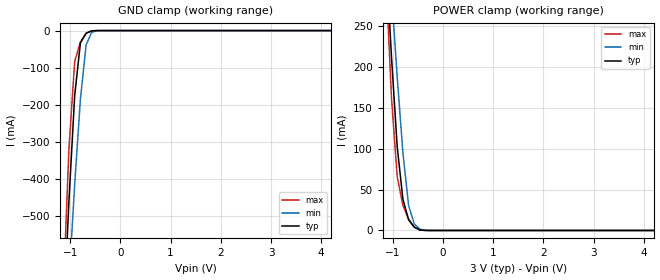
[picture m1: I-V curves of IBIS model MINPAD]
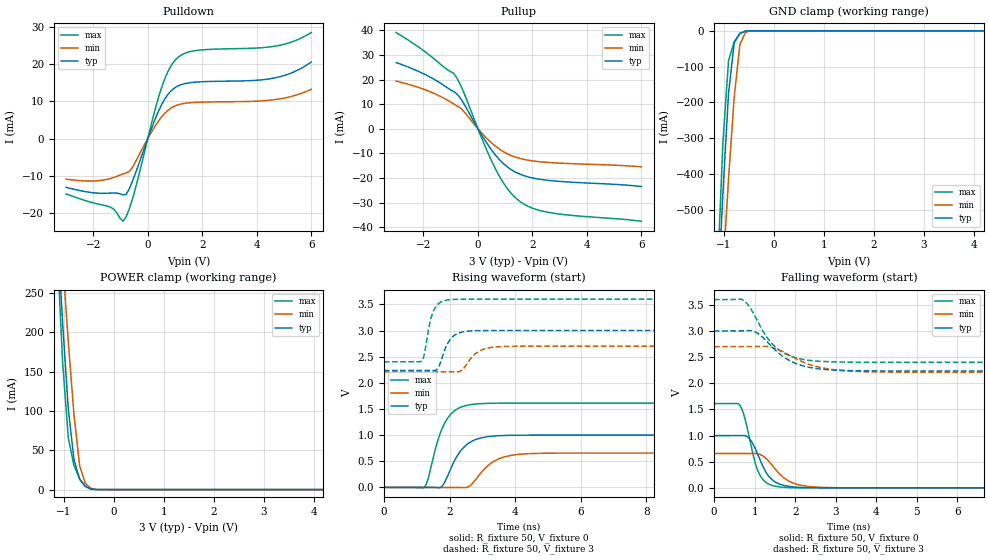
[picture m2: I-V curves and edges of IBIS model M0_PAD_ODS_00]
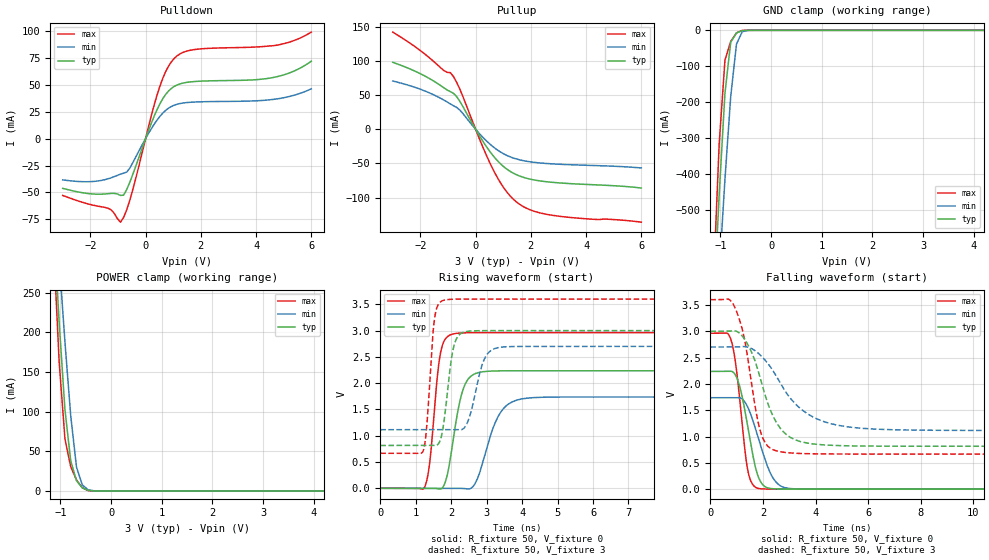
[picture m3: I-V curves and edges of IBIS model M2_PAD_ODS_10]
| Created by SiliconSmart  O-2018.09-SP2-3
[IBIS Ver]   4.0
[File Name]   as34b32bc_3p0_rev1p4.ibs
[File Rev]   1.4
[Date]   Thursday Mar 21 2024
|[Source]   Avalanche Team
|[Notes]   Generated IBIS models from Silicon Smart
|[Rev 1.0]  Initial Release based on extracted netlist
|   Characterization
|[Rev 1.1]  Recharacterization with Hspice, run in high accuracy mode
|[Rev 1.2]  Recharacterization with Hspice, parameters aligned with
|   datasheet
|[Rev 1.3]  Recharacterization with Hspice, run with updated VIH/VIL
|   in parallel with datasheet rev X.7
|[Rev 1.4]  Update the pin to the package pinout assignment
|[Disclaimer]   THE MODEL LIBRARIES ARE PROVIDED AS IS.
|[Copyright]   Copyright 2019, Avalanche Technology., All Rights Reserved
[Component]   AS304GB32_BGA
[Manufacturer] Avalanche Technology
| CONTENT :
| This file contains IBIS MODEL for PSRAM device
| AS304GB32
| USAGE :
| The models are derived for the 2.7V to 3.6V I/O Operation.
| Temperatures for model generation: typ: 25, max: -40, min: 125
| Voltages : typ: 3.0V, min: 2.7V, max: 3.6V
| PACKAGES SUPPORTED :
| 142-ball FBGA (15mm x 17mm)
| VERIFICATION
| Errors  : 0
| Warnings: 16
| All warnings due to non-monotonic data:
[Package]
R_pkg 0   0   0
L_pkg 0   0   0
C_pkg 0   0   0
[Pin]   signal_name   model_name   R_pin   L_pin   C_pin
P8   E#   MINPAD   0.254	7.307E-9	1.178E-12
P7   G#   MINPAD   0.243	7.052E-9	1.094E-12
J2   CR#   MINPAD   0.547	10.386E-9	1.789E-12
K3   PG#   MINPAD   0.451	10.329E-9	1.676E-12
M8   W#   MINPAD   0.377	9.020E-9	1.417E-12
M2   ADDR_26   MINPAD   0.425	9.037E-9	1.604E-12
L4   ADDR_25   MINPAD   0.419	9.644E-9	1.527E-12
K13   ADDR_24   MINPAD   0.495	9.978E-9	1.745E-12
M3   ADDR_23   MINPAD   0.371	9.313E-9	1.466E-12
L3   ADDR_22   MINPAD   0.412	9.753E-9	1.540E-12
M7   ADDR_21   MINPAD   0.368	8.765E-9	1.384E-12
P12   ADDR_20   MINPAD   0.287	8.287E-9	1.639E-12
L12   ADDR_19   MINPAD   0.424	10.320E-9	1.620E-12
N11   ADDR_18   MINPAD   0.338	8.691E-9	1.470E-12
N6   ADDR_17   MINPAD   0.309	8.196E-9	1.279E-12
P6   ADDR_16   MINPAD   0.256	7.462E-9	1.204E-12
L13   ADDR_15   MINPAD   0.463	10.719E-9	1.740E-12
M13   ADDR_14   MINPAD   0.421	10.290E-9	1.689E-12
P10   ADDR_13   MINPAD   0.262	7.671E-9	1.349E-12
N10   ADDR_12   MINPAD   0.340	8.540E-9	1.360E-12
M12   ADDR_11   MINPAD   0.402	9.876E-9	1.604E-12
N13   ADDR_10   MINPAD   0.399	9.819E-9	1.696E-12
L11   ADDR_9   MINPAD   0.443	9.732E-9	1.569E-12
M11   ADDR_8   MINPAD   0.436	9.682E-9	1.671E-12
P5   ADDR_7   MINPAD   0.253	7.464E-9	1.277E-12
P3   ADDR_6   MINPAD   0.279	8.031E-9	1.557E-12
N5   ADDR_5   MINPAD   0.313	8.320E-9	1.359E-12
N4   ADDR_4   MINPAD   0.329	8.138E-9	1.428E-12
M4   ADDR_3   MINPAD   0.379	8.543E-9	1.406E-12
N2   ADDR_2   MINPAD   0.378	9.572E-9	1.637E-12
N9   ADDR_1   MINPAD   0.315	8.416E-9	1.305E-12
M9   ADDR_0   MINPAD   0.403	9.225E-9	1.473E-12
E2   DQ_31   MIOPAD   0.365	8.798E-9	1.454E-12
F2   DQ_30   MIOPAD   0.418	9.057E-9	1.576E-12
D2   DQ_29   MIOPAD   0.358	8.697E-9	1.520E-12
E3   DQ_28   MIOPAD   0.348	8.812E-9	1.441E-12
E12   DQ_27   MIOPAD   0.327	8.506E-9	1.443E-12
D10   DQ_26   MIOPAD   0.309	7.715E-9	1.264E-12
C9   DQ_25   MIOPAD   0.279	7.395E-9	1.219E-12
C7   DQ_24   MIOPAD   0.252	6.802E-9	1.108E-12
G4   DQ_23   MIOPAD   0.455	10.071E-9	1.775E-12
G3   DQ_22   MIOPAD   0.457	10.100E-9	1.750E-12
F13   DQ_21   MIOPAD   0.377	9.387E-9	1.566E-12
D13   DQ_20   MIOPAD   0.295	8.231E-9	1.460E-12
C10   DQ_19   MIOPAD   0.293	7.553E-9	1.298E-12
E8   DQ_18   MIOPAD   0.393	8.323E-9	1.436E-12
F6   DQ_17   MIOPAD   0.425	8.913E-9	1.517E-12
E5   DQ_16   MIOPAD   0.379	8.982E-9	1.460E-12
E13   DQ_15   MIOPAD   0.363	8.555E-9	1.474E-12
G11   DQ_14   MIOPAD   0.475	9.536E-9	1.630E-12
E10   DQ_13   MIOPAD   0.404	8.563E-9	1.453E-12
F9   DQ_12   MIOPAD   0.409	9.347E-9	1.513E-12
C8   DQ_11   MIOPAD   0.257	6.782E-9	1.111E-12
C6   DQ_10   MIOPAD   0.238	7.000E-9	1.114E-12
D6   DQ_9   MIOPAD   0.292	7.776E-9	1.248E-12
D4   DQ_8   MIOPAD   0.305	7.782E-9	1.343E-12
G12   DQ_7   MIOPAD   0.502	10.055E-9	1.687E-12
C12   DQ_6   MIOPAD   0.275	7.857E-9	1.346E-12
D11   DQ_5   MIOPAD   0.286	7.835E-9	1.360E-12
D9   DQ_4   MIOPAD   0.306	8.035E-9	1.299E-12
E7   DQ_3   MIOPAD   0.384	8.178E-9	1.375E-12
C5   DQ_2   MIOPAD   0.231	6.786E-9	1.150E-12
D5   DQ_1   MIOPAD   0.307	7.698E-9	1.346E-12
C3   DQ_0   MIOPAD   0.267	7.420E-9	1.241E-12
G13   INT#   MIOPAD   0.480	10.704E-9	1.759E-12
F10   VSSIO   GND   NA   NA   NA
L10   VSSIO   GND   NA   NA   NA
E9   VSSIO   GND   NA   NA   NA
L9   VSSIO   GND   NA   NA   NA
F8   VSSIO   GND   NA   NA   NA
L8   VSSIO   GND   NA   NA   NA
F7   VSSIO   GND   NA   NA   NA
L7   VSSIO   GND   NA   NA   NA
E6   VSSIO   GND   NA   NA   NA
L6   VSSIO   GND   NA   NA   NA
G5   VSSIO   GND   NA   NA   NA
A14   VSS   GND   NA   NA   NA
B14   VSS   GND   NA   NA   NA
C14   VSS   GND   NA   NA   NA
H13   VSS   GND   NA   NA   NA
R14   VSS   GND   NA   NA   NA
T14   VSS   GND   NA   NA   NA
A13   VSS   GND   NA   NA   NA
T13   VSS   GND   NA   NA   NA
A12   VSS   GND   NA   NA   NA
G10   VSS   GND   NA   NA   NA
H10   VSS   GND   NA   NA   NA
J10   VSS   GND   NA   NA   NA
K10   VSS   GND   NA   NA   NA
F5   VSS   GND   NA   NA   NA
L5   VSS   GND   NA   NA   NA
A2   VSS   GND   NA   NA   NA
T2   VSS   GND   NA   NA   NA
A1   VSS   GND   NA   NA   NA
B1   VSS   GND   NA   NA   NA
R1   VSS   GND   NA   NA   NA
T1   VSS   GND   NA   NA   NA
F12   VCCIO   POWER   NA   NA   NA
J12   VCCIO   POWER   NA   NA   NA
E11   VCCIO   POWER   NA   NA   NA
M10   VCCIO   POWER   NA   NA   NA
D8   VCCIO   POWER   NA   NA   NA
N8   VCCIO   POWER   NA   NA   NA
D7   VCCIO   POWER   NA   NA   NA
N7   VCCIO   POWER   NA   NA   NA
M5   VCCIO   POWER   NA   NA   NA
E4   VCCIO   POWER   NA   NA   NA
F3   VCCIO   POWER   NA   NA   NA
J3   VCCIO   POWER   NA   NA   NA
C13   VCC   POWER   NA   NA   NA
P13   VCC   POWER   NA   NA   NA
D12   VCC   POWER   NA   NA   NA
N12   VCC   POWER   NA   NA   NA
C11   VCC   POWER   NA   NA   NA
F11   VCC   POWER   NA   NA   NA
H11   VCC   POWER   NA   NA   NA
J11   VCC   POWER   NA   NA   NA
K11   VCC   POWER   NA   NA   NA
P11   VCC   POWER   NA   NA   NA
C4   VCC   POWER   NA   NA   NA
F4   VCC   POWER   NA   NA   NA
H4   VCC   POWER   NA   NA   NA
J4   VCC   POWER   NA   NA   NA
K4   VCC   POWER   NA   NA   NA
P4   VCC   POWER   NA   NA   NA
D3   VCC   POWER   NA   NA   NA
N3   VCC   POWER   NA   NA   NA
C2   VCC   POWER   NA   NA   NA
P2   VCC   POWER   NA   NA   NA
| IOPAD
[Model Selector] MIOPAD
| Model Description
M0_PAD_ODS_00   ODS_00
M1_PAD_ODS_01   ODS_01
M2_PAD_ODS_10   ODS_10
M3_PAD_ODS_11   ODS_11
| Models and submodels in the file (5): MINPAD (Input), M0_PAD_ODS_00 (I/O), M2_PAD_ODS_10 (I/O), M1_PAD_ODS_01 (I/O), M3_PAD_ODS_11 (I/O)
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[Model] MINPAD
Model_type Input
Enable   Active-High
Vinl  =  0.8
Vinh  =  2.2
| Capacitance  typ   min   max
C_comp   6.130524e-12   5.673711e-12   6.587901e-12
| Variables   typ   min   max
[GND Clamp Reference]   0   0   0
[POWER Clamp Reference]   3   2.7   3.6
[Pulldown Reference]   0   0   0
[Pullup Reference]   3   2.7   3.6
[Temperature Range]   25   125   -40
[Voltage Range]   3   2.7   3.6
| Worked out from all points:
|   GND clamp passes 1 mA (typ) near -0.57 V on its own axis
|   POWER clamp passes 1 mA (typ) near -0.47 V on its own axis
[GND Clamp]
| Voltage   I(typ)   I(min)   I(max)
-3V       -6.848A    -5.961A    -8.2A
-1.138V   -783.9mA   -953.3mA   -701.6mA
-1.024V   -456.3mA   -675.8mA   -315.2mA
-910.3mV  -174.6mA   -413.8mA   -83.05mA
-796.6mV  -33.06mA   -184.3mA   -30.65mA
-682.8mV  -7.331mA   -38.2mA    -7.056mA
-569mV    -712.9uA   -3.879mA   -286.4uA
-455.2mV  -15.31uA   -289.9uA   -1.605uA
6V        0A         0A         0A
[POWER Clamp]
| Voltage   I(typ)   I(min)   I(max)
-3V       2.695A     2.364A     3.234A
-1.138V   339.1mA    399.9mA    313.8mA
-1.024V   212.3mA    291.5mA    162.2mA
-910.3mV  102.5mA    187.9mA    65.61mA
-796.6mV  38.13mA    95.01mA    30.53mA
-682.8mV  12.94mA    30.26mA    13.87mA
-569mV    3.981mA    7.764mA    4.118mA
-455.2mV  618.9uA    1.561mA    450.1uA
-227.6mV  142.3nA    9.251uA    10.37nA
6V        0A         0A         0A
[Model] M0_PAD_ODS_00
Model_type I/O
Enable   Active-High
Vinl  =  0.8
Vinh  =  2.2
Vmeas =  1.5
Cref  =  30e-12
| Capacitance  typ   min   max
C_comp   6.128805e-12   5.681079e-12   6.591827e-12
| Variables   typ   min   max
[GND Clamp Reference]   0   0   0
[POWER Clamp Reference]   3   2.7   3.6
[Pulldown Reference]   0   0   0
[Pullup Reference]   3   2.7   3.6
[Temperature Range]   25   125   -40
[Voltage Range]   3   2.7   3.6
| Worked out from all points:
|   slope of the pulldown table from 0 to 0.45 V, typ, clamps not added: 54.7 ohm
|   slope of the pullup table from 0 to 0.45 V, typ, clamps not added: 57.3 ohm
|   GND clamp passes 1 mA (typ) near -0.57 V on its own axis
|   POWER clamp passes 1 mA (typ) near -0.47 V on its own axis
|   falling waveform, R_fixture 50, V_fixture 0: 20-80 % time 391ps typ, 511ps min, 310ps max; typ from 1 V to 0 V
|   falling waveform, R_fixture 50, V_fixture 3: 20-80 % time 746ps typ, 889ps min, 639ps max; typ from 3 V to 2.23 V
|   rising waveform, R_fixture 50, V_fixture 0: 20-80 % time 564ps typ, 658ps min, 498ps max; typ from 0 V to 1 V
|   rising waveform, R_fixture 50, V_fixture 3: 20-80 % time 320ps typ, 421ps min, 242ps max; typ from 2.23 V to 3 V
[GND Clamp]
| Voltage   I(typ)   I(min)   I(max)
-3V       -6.848A    -5.961A    -8.2A
-1.138V   -783.9mA   -953.3mA   -701.6mA
-1.024V   -456.3mA   -675.8mA   -315.2mA
-910.3mV  -174.6mA   -413.8mA   -83.06mA
-796.6mV  -33.06mA   -184.3mA   -30.65mA
-682.8mV  -7.332mA   -38.2mA    -7.06mA
-569mV    -713uA     -3.879mA   -286.8uA
-455.2mV  -15.31uA   -289.9uA   -1.608uA
6V        0A         0A         0A
[POWER Clamp]
| Voltage   I(typ)   I(min)   I(max)
-3V       2.695A     2.364A     3.234A
-1.138V   339.1mA    399.9mA    313.8mA
-1.024V   212.3mA    291.5mA    162.2mA
-910.3mV  102.5mA    187.9mA    65.61mA
-796.6mV  38.13mA    95.01mA    30.53mA
-682.8mV  12.94mA    30.26mA    13.87mA
-569mV    3.981mA    7.764mA    4.118mA
-455.2mV  618.9uA    1.561mA    450.1uA
-227.6mV  142.3nA    9.251uA    10.37nA
6V        0A         0A         0A
[Pulldown]
| Voltage   I(typ)   I(min)   I(max)
-3V       -13.11mA   -10.91mA   -14.87mA
-1.366V   -14.66mA   -10.71mA   -18.44mA
-910.3mV  -15.13mA   -9.525mA   -22.23mA
-796.6mV  -15.02mA   -9.239mA   -20.99mA
-569mV    -11.56mA   -7.817mA   -16.37mA
206.9mV   4.069mA    2.602mA    6.097mA
517.2mV   9.226mA    5.888mA    13.93mA
724.1mV   11.7mA     7.479mA    17.77mA
1.034V    13.84mA    8.867mA    21.28mA
1.759V    15.14mA    9.703mA    23.62mA
4.614V    16.21mA    10.4mA     24.74mA
6V        20.54mA    13.21mA    28.45mA
[Pullup]
| Voltage   I(typ)   I(min)   I(max)
-3V       26.89mA    19.37mA    39.1mA
-1.821V   21.37mA    15.34mA    30.28mA
-910.3mV  15.2mA     10.23mA    22.74mA
-796.6mV  14.37mA    9.461mA    21.03mA
-569mV    11.16mA    7.659mA    16.04mA
206.9mV   -3.805mA   -2.558mA   -5.667mA
620.7mV   -10.37mA   -6.883mA   -15.82mA
1.034V    -15.12mA   -9.936mA   -23.64mA
1.552V    -18.5mA    -12.1mA    -29.65mA
2.069V    -20.15mA   -13.16mA   -32.55mA
2.69V     -21.11mA   -13.77mA   -34.19mA
6V        -23.51mA   -15.49mA   -37.63mA
[Ramp]
dV/dt_r   0.599879/0.564127n  0.393696/0.658178n  0.967082/0.498225n
dV/dt_f   0.45937/0.745634n  0.294233/0.889277n  0.719381/0.63933n
R_load = 50
[Falling Waveform]
R_fixture = 50
V_fixture = 0
V_fixture_min = 0
V_fixture_max = 0
| Time   V(typ)   V(min)   V(max)
0s        999.8mV    656.2mV    1.612V
634.8ps   1.001V     656.7mV    1.579V
867ps     945.1mV    656.9mV    971.6mV
1.014ns   753.5mV    657.3mV    480.2mV
1.125ns   552.1mV    642.6mV    251.3mV
1.359ns   214.2mV    499.7mV    69.66mV
1.655ns   62mV       237.1mV    14.65mV
2.145ns   8.265mV    48.76mV    1.268mV
2.985ns   772.1uV    3.26mV     186.7uV
21.88ns   34.45nV    448.9nV    -1.236uV
[Falling Waveform]
R_fixture = 50
V_fixture = 3
V_fixture_min = 2.7
V_fixture_max = 3.6
| Time   V(typ)   V(min)   V(max)
0s        3V         2.7V       3.6V
723.6ps   3.001V     2.701V     3.588V
897.7ps   3.007V     2.701V     3.434V
1.077ns   2.954V     2.703V     3.182V
1.304ns   2.8V       2.704V     2.878V
1.554ns   2.602V     2.655V     2.666V
2.021ns   2.377V     2.469V     2.486V
2.562ns   2.278V     2.313V     2.422V
4.529ns   2.235V     2.212V     2.401V
21.88ns   2.234V     2.21V      2.401V
[Rising Waveform]
R_fixture = 50
V_fixture = 0
V_fixture_min = 0
V_fixture_max = 0
| Time   V(typ)   V(min)   V(max)
0s        22.43nV    350.8nV    65.75nV
1.224ns   -348.6uV   -367.6uV   -154.8uV
1.341ns   -381.9uV   -402.7uV   154.3mV
1.719ns   -2.278mV   -516.6uV   1.04V
1.893ns   150.9mV    -568.8uV   1.276V
2.335ns   696mV      -2.644mV   1.531V
2.813ns   918.7mV    161.1mV    1.596V
3.412ns   985.1mV    518.7mV    1.61V
4.362ns   998.9mV    643.3mV    1.611V
21.88ns   999.8mV    656.2mV    1.612V
[Rising Waveform]
R_fixture = 50
V_fixture = 3
V_fixture_min = 2.7
V_fixture_max = 3.6
| Time   V(typ)   V(min)   V(max)
0s        2.234V     2.21V      2.401V
1.143ns   2.235V     2.21V      2.412V
1.221ns   2.235V     2.21V      2.521V
1.528ns   2.236V     2.21V      3.397V
1.668ns   2.302V     2.21V      3.516V
1.984ns   2.797V     2.211V     3.588V
2.353ns   2.966V     2.229V     3.599V
2.966ns   2.998V     2.625V     3.6V
3.626ns   3V         2.694V     3.6V
21.88ns   3V         2.7V       3.6V
[Model] M2_PAD_ODS_10
Model_type I/O
Enable   Active-High
Vinl  =  0.8
Vinh  =  2.2
Vmeas =  1.5
Cref  =  30e-12
| Capacitance  typ   min   max
C_comp   6.128805e-12   5.681079e-12   6.591827e-12
| Variables   typ   min   max
[GND Clamp Reference]   0   0   0
[POWER Clamp Reference]   3   2.7   3.6
[Pulldown Reference]   0   0   0
[Pullup Reference]   3   2.7   3.6
[Temperature Range]   25   125   -40
[Voltage Range]   3   2.7   3.6
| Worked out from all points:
|   slope of the pulldown table from 0 to 0.45 V, typ, clamps not added: 15.7 ohm
|   slope of the pullup table from 0 to 0.45 V, typ, clamps not added: 15.7 ohm
|   GND clamp passes 1 mA (typ) near -0.57 V on its own axis
|   POWER clamp passes 1 mA (typ) near -0.47 V on its own axis
|   falling waveform, R_fixture 50, V_fixture 0: 20-80 % time 504ps typ, 687ps min, 384ps max; typ from 2.24 V to 0 V
|   falling waveform, R_fixture 50, V_fixture 3: 20-80 % time 929ps typ, 1.5ns min, 599ps max; typ from 3 V to 0.815 V
|   rising waveform, R_fixture 50, V_fixture 0: 20-80 % time 347ps typ, 518ps min, 240ps max; typ from 0 V to 2.24 V
|   rising waveform, R_fixture 50, V_fixture 3: 20-80 % time 237ps typ, 342ps min, 175ps max; typ from 0.815 V to 3 V
[GND Clamp]
| Voltage   I(typ)   I(min)   I(max)
-3V       -6.848A    -5.961A    -8.2A
-1.138V   -783.9mA   -953.3mA   -701.6mA
-1.024V   -456.3mA   -675.8mA   -315.2mA
-910.3mV  -174.6mA   -413.8mA   -83.06mA
-796.6mV  -33.06mA   -184.3mA   -30.65mA
-682.8mV  -7.332mA   -38.2mA    -7.06mA
-569mV    -713uA     -3.879mA   -286.8uA
-455.2mV  -15.31uA   -289.9uA   -1.608uA
6V        0A         0A         0A
[POWER Clamp]
| Voltage   I(typ)   I(min)   I(max)
-3V       2.695A     2.364A     3.234A
-1.138V   339.1mA    399.9mA    313.8mA
-1.024V   212.3mA    291.5mA    162.2mA
-910.3mV  102.5mA    187.9mA    65.61mA
-796.6mV  38.13mA    95.01mA    30.53mA
-682.8mV  12.94mA    30.26mA    13.87mA
-569mV    3.981mA    7.764mA    4.118mA
-455.2mV  618.9uA    1.561mA    450.1uA
-227.6mV  142.3nA    9.251uA    10.37nA
6V        0A         0A         0A
[Pulldown]
| Voltage   I(typ)   I(min)   I(max)
-3V       -46.18mA   -38.31mA   -52.75mA
-1.366V   -51.15mA   -37.37mA   -64.58mA
-910.3mV  -52.72mA   -33.03mA   -77.58mA
-796.6mV  -52.54mA   -32.1mA    -73.2mA
-569mV    -40.41mA   -27.32mA   -57.03mA
206.9mV   14.21mA    9.09mA     21.22mA
517.2mV   32.23mA    20.57mA    48.54mA
724.1mV   40.88mA    26.13mA    61.99mA
1.034V    48.37mA    30.99mA    74.35mA
1.759V    52.94mA    33.91mA    82.6mA
4.614V    56.68mA    36.35mA    86.18mA
6V        71.86mA    46.21mA    98.85mA
[Pullup]
| Voltage   I(typ)   I(min)   I(max)
-3V       97.9mA     70.56mA    142mA
-1.821V   77.5mA     55.73mA    109.4mA
-910.3mV  54.96mA    36.99mA    82.75mA
-796.6mV  52.39mA    34.26mA    76.82mA
-569mV    40.81mA    28mA       58.57mA
103.4mV   -7.085mA   -4.779mA   -10.5mA
620.7mV   -37.92mA   -25.16mA   -57.78mA
1.034V    -55.27mA   -36.32mA   -86.42mA
1.552V    -67.66mA   -44.23mA   -108.4mA
2.069V    -73.7mA    -48.1mA    -119.1mA
2.793V    -77.6mA    -50.61mA   -125.8mA
6V        -85.91mA   -56.55mA   -135.8mA
[Ramp]
dV/dt_r   1.34189/0.346748n  1.04234/0.518069n  1.77705/0.239679n
dV/dt_f   1.31107/0.92907n  0.951014/1.49863n  1.76015/0.599415n
R_load = 50
[Falling Waveform]
R_fixture = 50
V_fixture = 0
V_fixture_min = 0
V_fixture_max = 0
| Time   V(typ)   V(min)   V(max)
0s        2.236V     1.737V     2.962V
796.3ps   2.239V     1.738V     2.824V
924.1ps   2.193V     1.738V     2.522V
1.085ns   2.01V      1.739V     1.875V
1.409ns   1.233V     1.573V     401.1mV
1.777ns   307.1mV    1.052V     19.7mV
2.019ns   71.09mV    658.7mV    4.314mV
2.393ns   7.349mV    206.2mV    1.223mV
3.049ns   893.7uV    10.99mV    368.5uV
21.88ns   -77.11nV   189.6nV    1.903uV
[Falling Waveform]
R_fixture = 50
V_fixture = 3
V_fixture_min = 2.7
V_fixture_max = 3.6
| Time   V(typ)   V(min)   V(max)
0s        3V         2.7V       3.6V
707.6ps   3.001V     2.7V       3.605V
978.1ps   3.003V     2.701V     3.404V
1.327ns   2.831V     2.707V     2.784V
1.897ns   2.114V     2.549V     1.115V
2.114ns   1.74V      2.433V     859.9mV
2.481ns   1.297V     2.172V     732.4mV
3.5ns     895.2mV    1.501V     676.3mV
5.249ns   823.2mV    1.182V     667mV
21.88ns   814.9mV    1.115V     666.4mV
[Rising Waveform]
R_fixture = 50
V_fixture = 0
V_fixture_min = 0
V_fixture_max = 0
| Time   V(typ)   V(min)   V(max)
0s        10.08nV    176.5nV    26.52nV
1.25ns    -105.4uV   -384.8uV   19.65mV
1.404ns   -118.4uV   -432.1uV   544.7mV
1.686ns   -15.2mV    -518.8uV   2.527V
2.052ns   905.8mV    -631.6uV   2.936V
2.289ns   1.777V     -1.627mV   2.955V
2.523ns   2.112V     -9.227mV   2.96V
3.377ns   2.234V     1.427V     2.961V
4.147ns   2.236V     1.715V     2.961V
21.88ns   2.236V     1.737V     2.962V
[Rising Waveform]
R_fixture = 50
V_fixture = 3
V_fixture_min = 2.7
V_fixture_max = 3.6
| Time   V(typ)   V(min)   V(max)
0s        814.9mV    1.115V     666.4mV
1.213ns   814.4mV    1.114V     714.9mV
1.309ns   814.4mV    1.114V     1.166V
1.522ns   814.3mV    1.114V     3.19V
1.804ns   1.301V     1.114V     3.581V
2.075ns   2.706V     1.114V     3.597V
2.466ns   2.987V     1.265V     3.6V
2.92ns    2.999V     2.436V     3.6V
3.426ns   2.999V     2.686V     3.6V
21.88ns   3V         2.7V       3.6V
